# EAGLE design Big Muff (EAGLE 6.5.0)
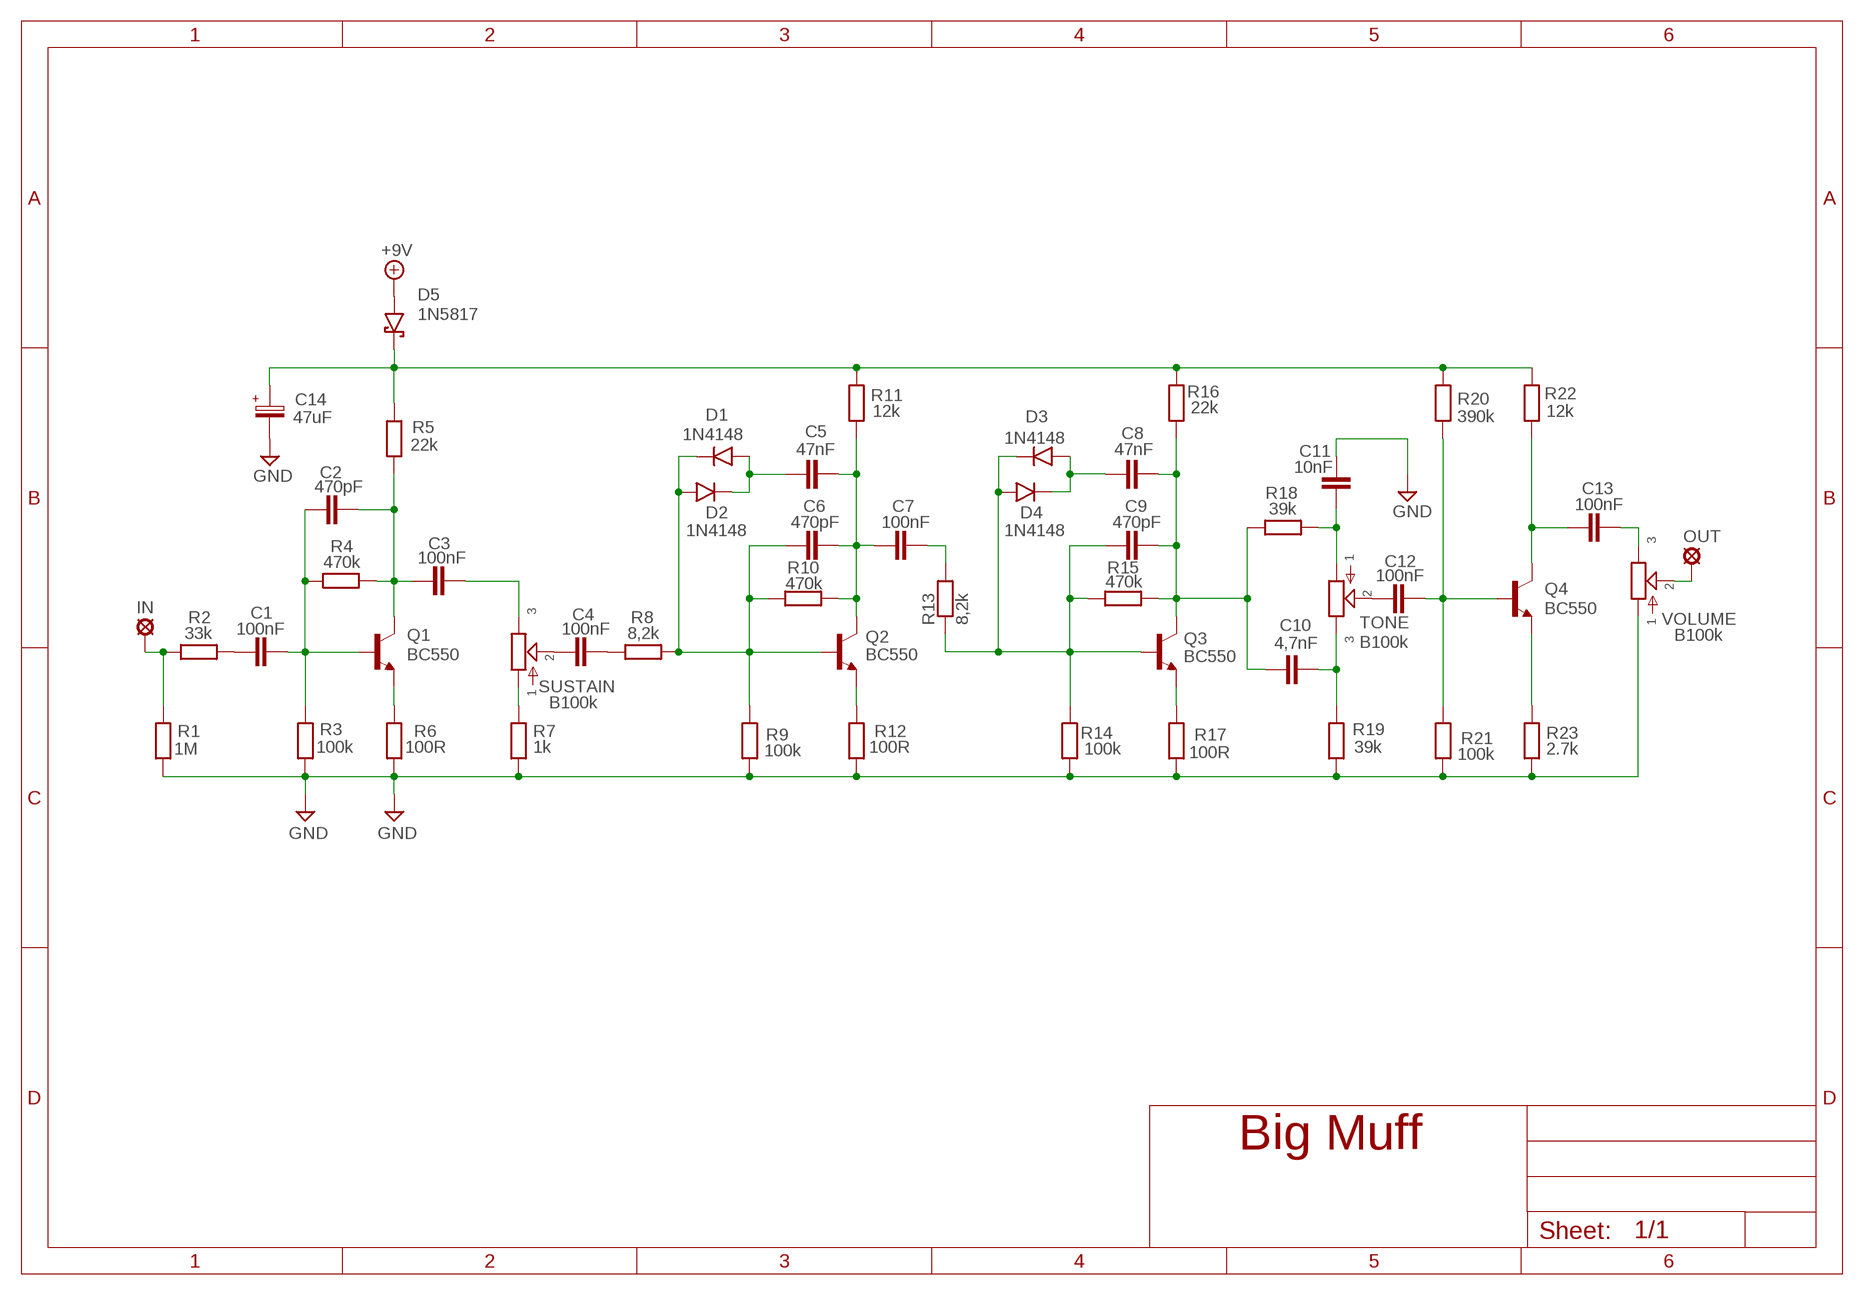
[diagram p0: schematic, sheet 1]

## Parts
+9V  +9V  +9V(T)1  [ROUND]
C1  100nF  100NF-220NF  [7,5MM]
C2  470pF  050X030_0251  [050X030_025]
C3  100nF  100NF-220NF  [7,5MM]
C4  100nF  100NF-220NF  [7,5MM]
C5  47nF  22NF-82NF"  [4,5MM]
C6  470pF  050X030_0251  [050X030_025]
C7  100nF  100NF-220NF  [7,5MM]
C8  47nF  22NF-82NF"  [4,5MM]
C9  470pF  050X030_0251  [050X030_025]
C10  4,7nF  1NF-15NF  [3,5MM]
C11  10nF  1NF-15NF  [3,5MM]
C12  100nF  100NF-220NF  [7,5MM]
C13  100nF  100NF-220NF  [7,5MM]
C14  47uF  050-EU1  [050_020_1]
D1  1N4148  1N4148-3  [DO35-3]
D2  1N4148  1N4148-3  [DO35-3]
D3  1N4148  1N4148-3  [DO35-3]
D4  1N4148  1N4148-3  [DO35-3]
D5  1N5817  [DO41-3]
GND  GND  GND(T)1  [ROUND]
GND1  GND  GND(T)1  [ROUND]
IN  MCS10B  [MCS10B]
OUT  MCS10B  [MCS10B]
Q1  BC550  [TO92-]
Q2  BC550  [TO92-]
Q3  BC550  [TO92-]
Q4  BC550  [TO92-]
R1  1M  6MM-EU3  [R0207/3]
R2  33k  6MM-EU3  [R0207/3]
R3  100k  6MM-EU3  [R0207/3]
R4  470k  6MM-EU3  [R0207/3]
R5  22k  6MM-EU3  [R0207/3]
R6  100R  6MM-EU3  [R0207/3]
R7  1k  6MM-EU3  [R0207/3]
R8  8,2k  6MM-EU3  [R0207/3]
R9  100k  6MM-EU3  [R0207/3]
R10  470k  6MM-EU3  [R0207/3]
R11  12k  6MM-EU3  [R0207/3]
R12  100R  6MM-EU3  [R0207/3]
R13  8,2k  6MM-EU3  [R0207/3]
R14  100k  6MM-EU3  [R0207/3]
R15  470k  6MM-EU3  [R0207/3]
R16  22k  6MM-EU3  [R0207/3]
R17  100R  6MM-EU3  [R0207/3]
R18  39k  6MM-EU3  [R0207/3]
R19  39k  6MM-EU3  [R0207/3]
R20  390k  6MM-EU3  [R0207/3]
R21  100k  6MM-EU3  [R0207/3]
R22  12k  6MM-EU3  [R0207/3]
R23  2.7k  6MM-EU3  [R0207/3]
SUSTAIN  B100k  POT-EU16MM  [16MM]
TONE  B100k  POT-EU16MM  [16MM]
VOLUME  B100k  POT-EU16MM  [16MM]

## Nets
+9V: +9V.1(+9V) D5.A
GND: C11.1 C14.- GND1.1(GND) GND.1(GND) R1.1 R3.1 R6.1 R7.1 R9.1 R12.1 R14.1 R17.1 R19.1 R21.1 R23.1 VOLUME.1
N$1: C1.P$1 R2.2
N$2: Q1.1(E) R6.2
N$3: C4.P$1 SUSTAIN.2
N$4: R7.2 SUSTAIN.1
N$5: C4.P$2 R8.1
N$6: Q2.1(E) R12.2
N$7: Q3.1(E) R17.2
N$8: C12.P$1 TONE.2
N$9: Q4.1(E) R23.2
N$10: C2.2 C3.P$1 Q1.3(C) R4.2 R5.1
N$11: C5.2 C6.2 C7.P$1 Q2.3(C) R10.2 R11.1
N$12: C8.2 C9.2 C10.1 Q3.3(C) R15.2 R16.1 R18.1
N$13: C13.P$1 Q4.3(C) R22.1
N$14: C1.P$2 C2.1 Q1.2(B) R3.2 R4.1
N$15: C6.1 D1.C D2.A Q2.2(B) R8.2 R9.2 R10.1
N$16: C12.P$2 Q4.2(B) R20.1 R21.2
N$17: C3.P$2 SUSTAIN.3
N$18: C7.P$2 R13.2
N$19: C9.1 D3.C D4.A Q3.2(B) R13.1 R14.2 R15.1
N$20: C11.2 R18.2 TONE.1
N$21: C5.1 D1.A D2.C
N$22: C8.1 D3.A D4.C
N$23: C10.2 R19.2 TONE.3
N$24: C13.P$2 VOLUME.3
N$25: IN.MP R1.2 R2.1
N$26: OUT.MP VOLUME.2
N$27: C14.+ D5.C R5.2 R11.2 R16.2 R20.2 R22.2

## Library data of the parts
+9V = gm-supply:+9V(T): +9V Voltage Supply
C1 C3 C4 C7 C12 C13 = Mylar Kondensaattorit:100NF-220NF: 100nF-220nF
C2 C6 C9 = Keraamiset kondensaattorit:050X030_025: 47 - 120pF
C5 C8 = Mylar Kondensaattorit:22NF-82NF: 22nF-82nF
C10 C11 = Mylar Kondensaattorit:1NF-15NF: 1nF-15nF
C14 = Elektrolyytit:050-EU
D1-D4 = Diodit:1N4148: Fast Switching Diode
D5 = Diodit:1N5817
GND GND1 = gm-supply:GND(T): Ground
IN OUT = Padit:MCS10B: SOLDER PAD
Q1-Q4 = Transistorit:BC550
R1-R23 = Vastukset:6MM-EU: 6mm Resistors (European schematic symbol)
SUSTAIN TONE VOLUME = gm-pots:POT-EU

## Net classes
0 default: width 0.406 mm

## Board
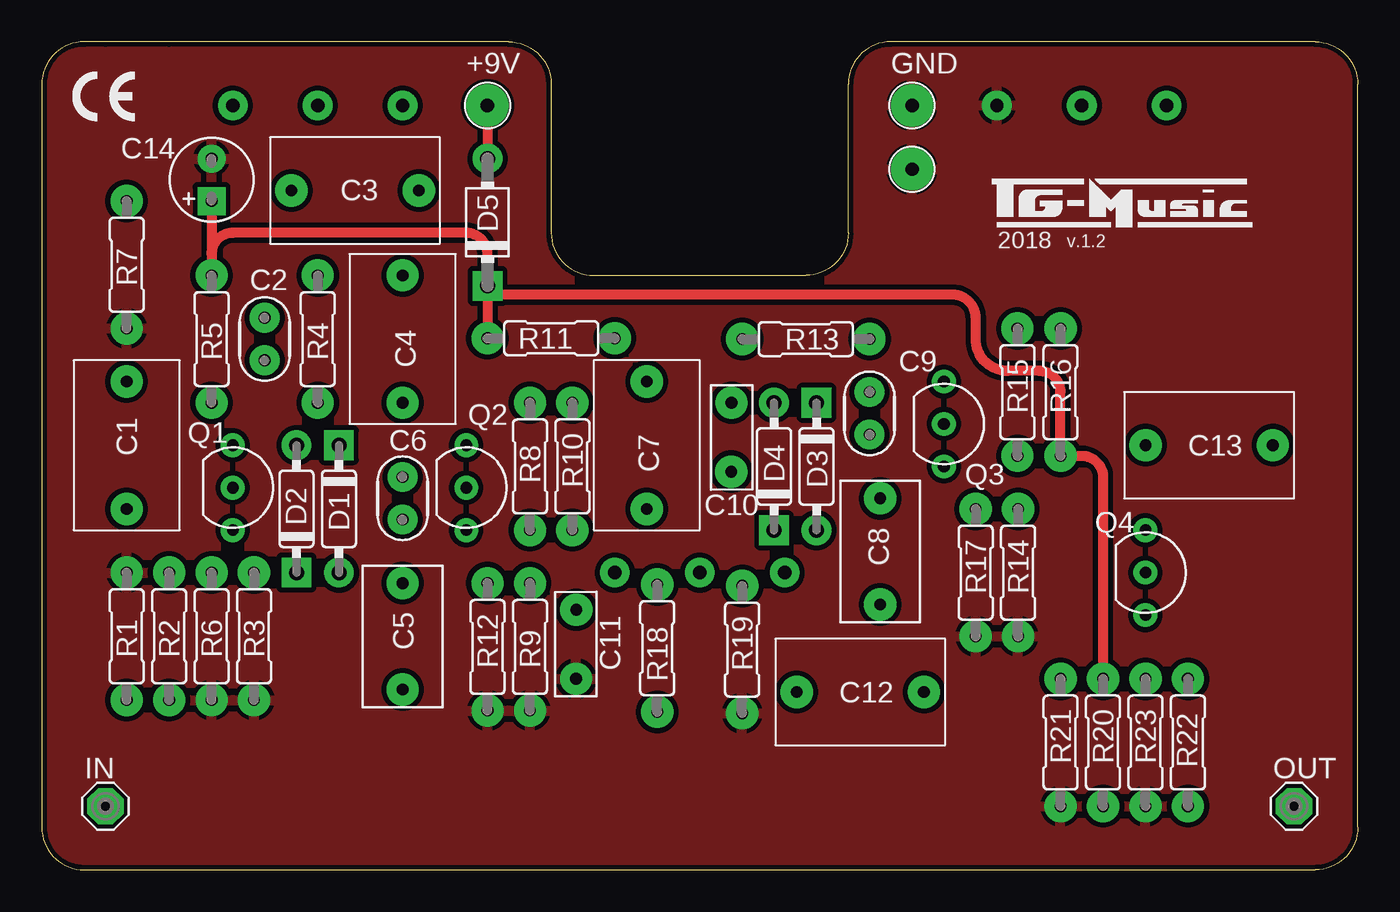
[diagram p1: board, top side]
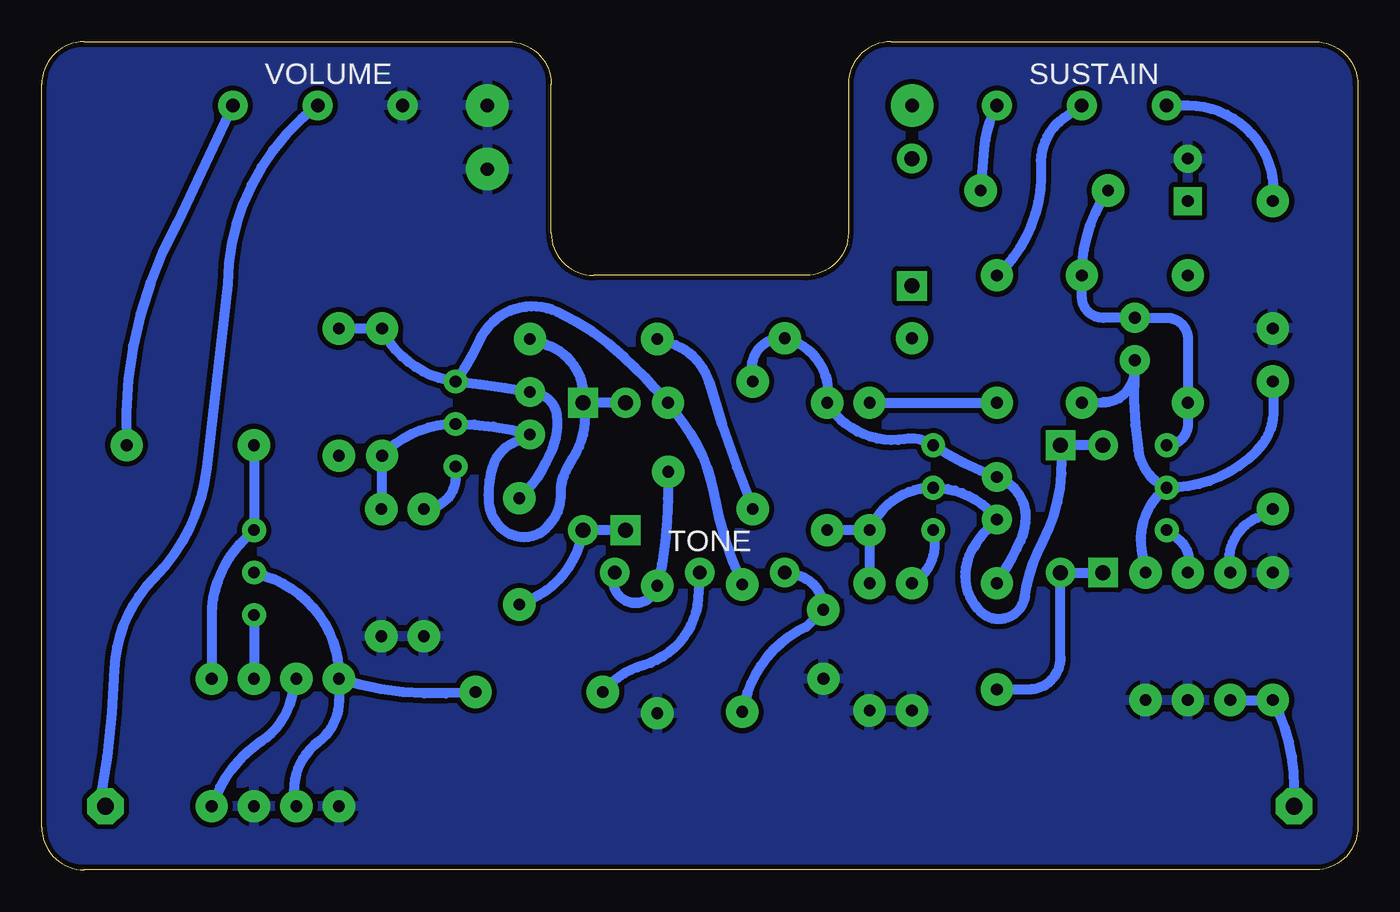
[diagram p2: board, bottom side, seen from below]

Size 78.74 x 49.53 mm. Coordinates in mm from the lower left corner, seen from the top.
Outline: 7.62,49.53 3.81,49.53
Outline: 78.74,2.54 78.74,46.99 arc90 76.2,49.53 50.8,49.53 arc90 48.26,46.99 48.26,38.1 arc-90 45.72,35.56 33.02,35.56 arc-90 30.48,38.1 30.48,46.99 arc90 27.94,49.53 2.54,49.53 arc90 0,46.99 0,2.54 arc90 2.54,0 76.2,0 arc90 78.74,2.54
Copper layers (1*16): Top 0.035mm / dielectric 1.5mm / Bottom 0.035mm
Design rules "ITEADstudio": minimum track width 10mil, minimum drill 12mil, track to track 12mil, track to pad 12mil, pad to pad 12mil, via to via 12mil, smd to smd 0mil, copper to edge 12mil, drill to drill 12mil, minimum pad ring 10mil, minimum via ring 6mil, stop-mask expansion 4mil, vias tented up to drill 100mil, thermal gap 10mil

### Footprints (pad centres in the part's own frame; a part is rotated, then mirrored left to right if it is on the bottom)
ROUND = drill 0.8 pad 2.54: 1 0,0
7,5MM = drill 0.7 pad 1.93: P$1 -3.81,0; P$2 3.81,0
050X030_025 = drill 0.7 pad 1.778: 1 -1.27,0; 2 1.27,0
4,5MM = drill 0.7 pad 1.93: 1 -3.175,0; 2 3.175,0
3,5MM = drill 0.7 pad 1.93: 1 -1.905,0; 2 2.221,-0.016
050_020_1 = drill 0.7 pad 1.676 square: + -1.27,0 | drill 0.7 pad 1.676: - 1.27,0
DO35-3 = drill 0.9 pad 1.778: A 3.81,0 | drill 0.9 pad 1.778 square: C -3.81,0
DO41-3 = drill 0.9 pad 1.778: A 3.81,0 | drill 0.9 pad 1.778 square: C -3.81,0
MCS10B = drill 1.016 pad 2.159 octagon: MP 0,0
TO92- = drill 0.7 pad 1.422: 1 2.54,0; 2 0,0; 3 -2.54,0
R0207/3 = drill 0.7 pad 1.93: 1 -3.81,0; 2 3.81,0
16MM = drill 0.8 pad 1.778: 1 5.08,0; 2 0,0; 3 -5.08,0

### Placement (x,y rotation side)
+9V  26.67,45.72 0 top
C1  5.08,25.4 90 top
C2  13.34,31.75 90 top
C3  18.74,40.63 0 top
C4  21.59,31.75 270 top
C5  21.59,13.97 90 top
C6  21.59,22.23 90 top
C7  36.2,25.4 270 top
C8  50.16,19.05 90 top
C9  49.53,27.3 90 top
C10  41.27,26.04 270 top
C11  31.96,13.34 90 top
C12  48.98,10.64 0 top
C13  69.85,25.4 0 top
C14  10.16,41.27 90 top
D1  17.78,21.59 270 top
D2  15.24,21.59 90 top
D3  46.35,24.13 270 top
D4  43.81,24.13 90 top
D5  26.67,38.73 90 top
GND  52.07,45.72 0 top
GND1  52.07,41.91 0 top
IN  3.81,3.81 0 top
OUT  74.93,3.81 0 top
Q1  11.43,22.86 270 top
Q2  25.4,22.86 270 top
Q3  53.98,26.67 270 top
Q4  66.04,17.78 270 top
R1  5.08,13.97 270 top
R2  7.62,13.97 90 top
R3  12.7,13.97 90 top
R4  16.51,31.75 90 top
R5  10.16,31.75 90 top
R6  10.16,13.97 90 top
R7  5.08,36.2 90 top
R8  29.21,24.13 270 top
R9  29.21,13.34 90 top
R10  31.75,24.13 90 top
R11  30.48,31.8 180 top
R12  26.67,13.34 90 top
R13  45.72,31.75 180 top
R14  58.42,17.78 90 top
R15  58.38,28.57 90 top
R16  60.96,28.57 270 top
R17  55.88,17.78 90 top
R18  36.82,13.26 270 top
R19  41.91,13.18 90 top
R20  63.5,7.62 90 top
R21  60.96,7.62 90 top
R22  68.58,7.62 270 top
R23  66.04,7.62 90 top
SUSTAIN  16.51,45.72 0 bottom
TONE  39.37,17.78 0 bottom
VOLUME  62.23,45.72 0 bottom

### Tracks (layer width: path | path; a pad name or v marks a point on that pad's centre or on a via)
+9V
  Top 0.61: +9V.1 D5.A
GND
  pour Bottom: 0,2.54 0,46.99 arc-90 2.54,49.53 27.94,49.53 arc-90 30.48,46.99 30.48,38.1 arc90 33.02,35.56 45.72,35.56 arc90 48.26,38.1 48.26,46.99 arc-90 50.8,49.53 76.2,49.53 arc-90 78.74,46.99 78.74,2.54 arc-90 76.2,0 2.54,0 arc-90
  pour Top: 0,2.54 0,46.99 arc-90 2.54,49.53 27.94,49.53 arc-90 30.48,46.99 30.48,38.1 arc90 33.02,35.56 45.72,35.56 arc90 48.26,38.1 48.26,46.99 arc-90 50.8,49.53 76.2,49.53 arc-90 78.74,46.99 78.74,2.54 arc-90 76.2,0 2.54,0 arc-90
N$1
  Bottom 0.61: C1.P$1 4.99,21.29 arc-103 R2.2
N$2
  Bottom 0.61: Q1.1 10.79,19.82 arc70 R6.2
N$3
  Bottom 0.61: SUSTAIN.2 17.59,44.96 arc-58 18.96,42.14 arc50 C4.P$1
N$4
  Bottom 0.61: SUSTAIN.1 10.16,45.72 arc97 R7.2
N$5
  Bottom 0.61: R8.1 C4.P$2
N$6
  Bottom 0.61: Q2.1 25.34,19.75 arc67 R12.2
N$7
  Bottom 0.61: Q3.1 53.98,23.5 arc90 R17.2
N$8
  Bottom 0.61: TONE.2 39.47,16.26 arc70 42.72,12.25 arc-35 C12.P$1
N$9
  Bottom 0.61: Q4.1 R23.2
N$10
  Bottom 0.61: Q1.3 arc-90 10.16,26.67 R5.1 10.16,31.75 arc-90 11.43,33.02 C2.2 15.24,33.02 arc90 16.51,34.29 R4.2 arc35 C3.P$1
N$11
  Bottom 0.61: C5.2 20.94,18.22 arc-7 20.18,19.68 arc-23 19.86,21.05 arc-34 20.23,22.4 arc-38 C6.2 arc14 Q2.3 arc-43 27.09,25.77 arc68 R10.2 31.75,27.99 arc-87 R11.1 arc-100 36.25,29.89 C7.P$1
N$12
  Bottom 0.61: R16.1 R15.2 | R15.2 arc90 R15.2 | C8.2 arc-18 48.82,23.91 arc-8 48.19,25.21 arc-29 47.93,27.21 arc-73 49.19,28.52 C9.2 arc-3 Q3.3 | Q3.3 arc58 R15.2 | Q3.3 arc-10 52.54,31.69 arc90 47.9,33.37 arc17 43.9,30.68 arc6 42.06,28.82 C10.1 40.38,26.76 arc27 38.55,22.57 arc-14 R18.1
N$13
  Bottom 0.61: C13.P$1 Q4.3 66.86,19.5 arc-43 68.56,15.14 68.56,12.49 R22.1
N$14
  Bottom 0.61: C1.P$2 5.04,27.62 arc47 6.1,25 arc46 Q1.2 | C2.1 13.37,29.57 | 13.37,29.57 arc-11 13.14,25.11 arc-58 Q1.2 | R4.1 15.21,27.97 arc-80 13.37,29.57 | R3.2 12.92,19.15 arc62 Q1.2
N$15
  Bottom 0.61: D2.A D1.C arc35 18.85,19.62 arc-20 19.91,16.36 arc125 22.56,15.44 arc46 23.48,17.56 arc32 23.01,19.28 arc12 22.19,20.34 C6.1 arc-53 Q2.2 arc-67 R8.2 | R8.2 R10.1 | R8.2 R9.2
N$16
  Bottom 0.61: R21.2 60.96,10.16 arc53 62.23,7.62 arc-69 R20.1 | Q4.2 65.36,17.57 arc74 R21.2 | C12.P$2 54.55,10.56 arc20 R21.2
N$17
  Bottom 0.61: C3.P$2 22.34,43.12 arc23 SUSTAIN.3
N$18
  Bottom 0.61: R13.2 41.09,31.49 arc56 38.83,29.18 arc-5 C7.P$2
N$19
  Bottom 0.61: D3.C arc47 46.94,24.66 arc-18 47.6,23.23 arc-18 47.68,22.56 arc55 48.72,20.31 arc66 50.78,20.12 arc58 52,21.98 arc21 51.76,24.12 arc46 50.59,25.5 C9.1 arc-16 Q3.2 arc-47 R15.1 58.42,24.77 R14.2 | D4.A D3.C | R13.1 48.55,31.42 arc78 D3.C
N$20
  Bottom 0.61: TONE.1 33.67,17.66 arc81 C11.2 33,14.54 arc-55 R18.2
N$21
  Bottom 0.61: D2.C D1.A 17.78,12.7 arc90 19.68,10.79 C5.1
N$22
  Bottom 0.61: D4.C D3.A arc57 49.41,16.22 C8.1
N$23
  Bottom 0.61: C10.2 41.27,22.23 arc13 R19.2 arc188 TONE.3
N$24
  Bottom 0.61: VOLUME.3 70.61,38.75 arc-32 C13.P$2
N$25
  Bottom 0.61: IN.MP 3.8,4.98 arc-29 R1.2 R2.1
N$26
  Bottom 0.61: VOLUME.2 62.31,45.66 arc-52 67.61,35.02 68.87,24.05 arc38 72.06,17.4 arc-43 74.39,12.01 arc8 75.24,4.19 75.24,4.12 OUT.MP
N$27
  Top 0.61: D5.C 26.67,36.83 arc90 25.4,38.1 11.43,38.1 arc90 10.16,36.83 | 10.16,36.83 R5.2 | R20.2 63.5,23.5 arc90 62.23,24.77 R16.2 60.96,28.57 arc90 59.69,29.84 57.78,29.84 arc-90 55.88,31.75 55.88,33.02 arc90 54.49,34.41 27.19,34.41 D5.C | C14.+ 10.16,36.83 | D5.C R11.2
  Bottom 0.61: R20.2 63.81,10.24 arc41 65.6,7.69 arc-36 R22.2

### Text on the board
tNames: 2018 | v.1.2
